TYPE ST_AlarmID :
(*报警的id号，swen*)
STRUCT
	(*系统*)
	EtherCATBusErr:					INT:=1;(*EtherCAT总线错误*)
	SystemLoading:					INT:=2;(*系统启动中*)
	EmergentStop:					INT:=3;(*急停按钮*)
	ProductChangeNeedSave:			INT:=4;
	ProductLoadingNoPowerOff:		INT:=5;
	AirPressLow:					INT:=6;(*气压低!*)
	Prushing:						INT:=7;(*暂停中*)
	NeedHoming:						INT:=8;(*开机前请先找原点*)
	IsHoming:						INT:=9;(*正在找原点*)
	AutoStoping:					INT:=10;(*自动停机中*)
	AutoStopImediery:				INT:=11;(*马上停机中*)
	AutoRuning:						INT:=12;(*设备运行中*)
	ComErrorVS:						INT:=13;(*视觉控制器通讯异常*)
	ServoError:						INT:=14;(*伺服出错*)
	ServoHwError:					INT:=15;(*伺服驱动器报错，硬件报错*)
	ServoLimit:						INT:=16;(*伺服驱动器限位到*)
	CycleTimeOut:					INT:=17;(*循环时间超时*)
	ModbusRtuError:					INT:=18;(*ModbusRtu总线错误*)
	RobotError1:					INT:=19;(*机器人错误*)
	RobotError2:					INT:=20;(*机器人错误*)
	StepServoError:					INT:=21;(*步进驱动器报错*)
	RobotSN_Error:					INT:=22;(*机器人序列号异常*)

	(*程序逻辑*)
	ClampVacuum:					INT:=26;(*机器人1真空吸取失败*)








	(*序列号*)
	Machime_SoftHwDif:				INT:=50;(*软硬件不匹配*)
	Machime_Alarm_NeedKey:			INT:=51;(*系统即将进入维护模式*)
	Machime_Stop_NeedKey:			INT:=52;(*系统已经进入维护模式*)

END_STRUCT
END_TYPE
